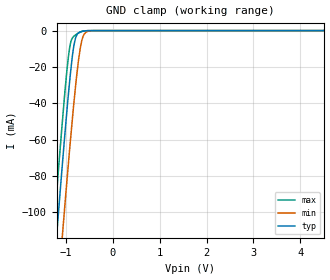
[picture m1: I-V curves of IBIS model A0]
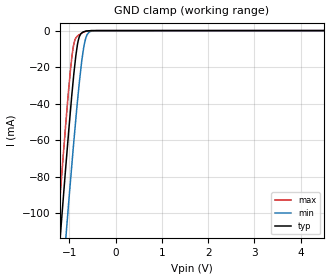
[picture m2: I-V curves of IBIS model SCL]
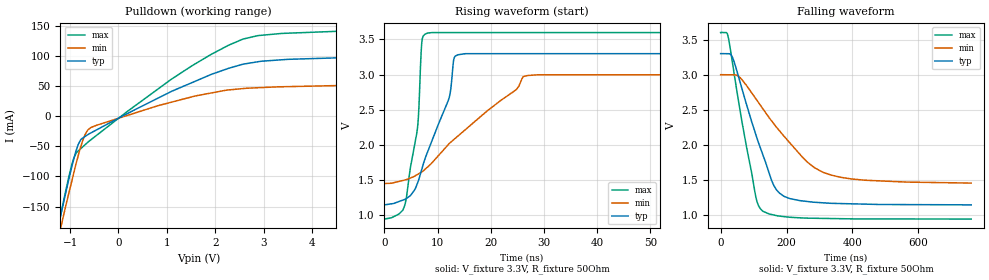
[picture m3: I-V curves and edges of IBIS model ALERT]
|Texas Instruments Incorporated
|Temperature and Supply System Monitors
|   SMBus interface
| Marketing part#   Digital Voltge  Analog Voltage   Package-type   #pins
|   Range   Range
|TMP512AIDG4   2.1V to 3.6V   3.0V to 26V   SO-14   14
|TMP512AIDRG4   2.1V to 3.6V   3.0V to 26V   SO-14   14
|TMP513AIDG4   2.1V to 3.6V   3.0V to 26V   SO-16   16
|TMP513AIDRG4   2.1V to 3.6V   3.0V to 26V   SO-16   16
|TMP513AIRSATG4   2.1V to 3.6V   3.0V to 26V   QFN-16   16
|TMP513AIRSARG4   2.1V to 3.6V   3.0V to 26V   QFN-16   16
[IBIS Ver]   4.0
[File name]   tmp512_3.ibs
[File Rev]   1.0
[Date]   04/14/2010
[Source]   Texas Instruments Incorporated.
   Analog-eLab, HPA
   12500 TI Blvd
   Dallas, TX -75243
   For Support e-mail: elab_ibis@list.ti.com
[Notes]   Revision History:
   1.0: 04/14/2010
   - Initial version of the model
   - Initial Model generated from simulations in TISPICED
   - Model not matched to measurements
   - Non-monotnic warnings - combined pulldown and pullup data
   The GPIO non-monotonic current delta is less than 1 mA in a
   full-scale range of ~95 mA. Given these conditions, these
   warnings are deemed insignificant.
   1.1: 04/18/2010 corrected spelling errors
[Disclaimer]
 This product is designed as an aid for customers of Texas Instruments.
 No warranties, either expressed or implied, with respect to this third
 party software (if any) or with respect to its fitness for any
 particular purpose is claimed by Texas Instruments or the author. The
 software (if any) is provided solely on an "as is" basis. The entire
 risk as to its quality and performance is with the customer
[Copyright] (C) Copyright 2009 Texas Instruments Incorporated.
   All rights reserved.
|   TMP512
[Component]   tmp512d   |SO-14
[Manufacturer] TI
[Package]
| variable   typ   min   max
R_pkg  0.069985   0.043420   0.089600
L_pkg  2.478174nH  1.695740nH  3.523510nH
C_pkg  0.468851pF  0.340100pF  0.678470pF
[Pin] signal_name  model_name  R_pin  L_pin C_pin
1   FILTER_C   TERM   0.04342  3.11995nH  0.67449pF
2   VP   POWER   0.08667  2.52082nH  0.46308pF
3   VINP   TERM   0.07721  2.16899nH  0.36364pF
4   VINM   TERM   0.05969  1.82032nH  0.34660pF
5   SDA   SDA   0.06085  1.85014nH  0.35048pF
6   SCL   SCL   0.08960  2.59142nH  0.46438pF
7   A0   A0   0.08471  3.52351nH  0.63150pF
8   DXP1   TERM   0.08391  3.50902nH  0.62842pF
9   DXN1   TERM   0.08732  2.54500nH  0.45919pF
10   DXP2   TERM   0.06400  1.91255nH  0.35199pF
11   DXN2   TERM   0.05307  1.69574nH  0.34010pF
12   GPIO   GPIO   0.06106  1.84901nH  0.34913pF
13   ALERT   ALERT   0.08484  2.48378nH  0.46244pF
14   GND   GND   0.04344  3.10418nH  0.6784pF
|   TMP513
[Component]   tmp513d   |SO-16
[Manufacturer] TI
[Package]
| variable   typ   min   max
R_pkg  0.065299   0.037330   0.101480
L_pkg  2.886102nH  1.773530nH  4.324090nH
C_pkg  0.858015pF  0.604310pF  1.222580pF
[Pin] signal_name  model_name  R_pin  L_pin C_pin
1   FILTER_C   TERM   0.03733  3.81993nH  1.22058pF
2   VP   POWER   0.06446  3.16263nH  0.96919pF
3   VINP   TERM   0.10148  2.80051nH  0.66655pF
4   VINM   TERM   0.07726  2.32345nH  0.63122pF
5   SDA   SDA   0.04983  1.78009nH  0.60589pF
6   SCL   SCL   0.07392  2.24087nH  0.64264pF
7   A0   A0   0.06334  3.16918nH  0.95352pF
8   DXP1   TERM   0.08068  4.32409nH  1.19594pF
9   DXN1   TERM   0.06968  4.10189nH  1.18926pF
10   DXP2   TERM   0.06456  3.19343nH  0.95660pF
11   DXN2   TERM   0.07197  2.20137nH  0.63879pF
12   DXP2   TERM   0.04946  1.77353nH  0.60431pF
13   DXN3   TERM   0.05950  1.96740nH  0.61338pF
14   GPIO   GPIO   0.08122  2.38171nH  0.64891pF
15   ALERT   ALERT   0.06271  3.12769nH  0.96888pF
16   GND   GND   0.03739  3.80986nH  1.22258pF
|   TMP513
[Component]   tmp513rsa   |QFN-16
[Manufacturer] TI
[Package]
| variable   typ   min   max
R_pkg  0.059859   0.031800   0.075880
L_pkg  1.070891nH  0.737920nH  1.352600nH
C_pkg  0.106648pF  0.097070pF  0.132860pF
[Pin] signal_name  model_name  R_pin  L_pin C_pin
1   VINP   TERM   0.07469  1.32940nH  0.11305pF
2   VINM   TERM   0.07588  1.35260nH  0.11568pF
3   SDA   SDA   0.06628  1.16760nH  0.10737pF
4   SCL   SCL   0.06192  1.08495nH  0.10230pF
5   A0   A0   0.05892  1.02585nH  0.09707pF
6   DXP1   TERM   0.06624  1.16590nH  0.10463pF
7   DXN1   TERM   0.05844  1.01645nH  0.09772pF
8   DXP2   TERM   0.06034  1.04942nH  0.09981pF
9   DXN2   TERM   0.06180  1.07436nH  0.10070pF
10   DXP3   TERM   0.06430  1.12203nH  0.10277pF
11   DXN3   TERM   0.06376  1.11165nH  0.10130pF
12   GPIO   GPIO   0.06338  1.10445nH  0.10153pF
13   ALERT   ALERT   0.05826  1.01150nH  0.09857pF
14   GND   GND   0.03196  0.73792nH  0.13286pF
15   FILTER_C   TERM   0.03180  0.73867nH  0.13120pF
16   VP   POWER   0.05978  1.04150nH  0.09980pF
|   TERM Model
[Model] TERM
Model_type Terminator
C_comp   1e-20   1e-20   1e-20
| variable   typ   min   max
[Voltage Range]   5.0V   3.3V   26V
[POWER Clamp Reference]  5.0V   3.3V   26V
[GND Clamp Reference]   0.0V   0.0V   0.0V
|Operating Temperature
[Temperature Range]   27   125   -40
| Models and submodels in the file (6): TERM (Terminator), A0 (Input), SCL (Input), ALERT (Open_drain), GPIO (I/O), SDA (I/O_open_drain)
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|   A0   3.3V digital input
[Model] A0
Model_type Input
Vinl = 0.8
Vinh = 2.1
|   typ   min   max
C_comp   1.3747800e-12   1.1549790e-12   1.6089250e-12
[Voltage Range]   3.3   3   3.6
[Temperature Range]   27   125   -40
[GND Clamp Reference]   0   0   0
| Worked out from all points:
|   GND clamp passes 1 mA (typ) near -0.72 V on its own axis
[GND Clamp]
|   Voltage   I(typ)   I(min)   I(max)
-3.3V     -841.9mA   -868mA     -829.4mA
-1.298V   -146.1mA   -184.7mA   -123.2mA
-1.247V   -129.3mA   -168mA     -106mA
-1.198V   -112.9mA   -152mA     -89.56mA
-1.089V   -77.76mA   -117mA     -54.11mA
-1.03V    -59.6mA    -98.77mA   -36.38mA
-922.3mV  -28.52mA   -65.93mA   -9.815mA
-828mV    -7.978mA   -39.34mA   -3.032mA
-706.6mV  -822.9uA   -11.99mA   -1.042mA
-612.5mV  -190.6uA   -2.027mA   -280.3uA
-420.7mV  -23.27uA   -24.62uA   -25.64uA
6.59V     0A         0A         0A
[POWER Clamp]
|   SCR cell for ESD function. Effects occurr above VDD x 2
|   Voltage   I(typ)   I(min)   I(max)
-3.3V     0A         0A         0A
0V        0A         0A         0A
6.6V      0A         0A         0A
|   SCL   3.3V digital input
[Model] SCL
Model_type Input
Vinl = 0.8
Vinh = 2.1
|   typ   min   max
C_comp   1.3747800e-12   1.1549790e-12   1.6089250e-12
[Voltage Range]   3.3   3   3.6
[Temperature Range]   27   125   -40
[GND Clamp Reference]   0   0   0
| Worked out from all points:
|   GND clamp passes 1 mA (typ) near -0.72 V on its own axis
[GND Clamp]
|   Voltage   I(typ)   I(min)   I(max)
-3.3V     -841.9mA   -868mA     -829.4mA
-1.268V   -136.1mA   -174.8mA   -113mA
-1.213V   -118mA     -156.9mA   -94.64mA
-1.172V   -104.6mA   -143.8mA   -81.14mA
-1.081V   -75.19mA   -114.5mA   -51.62mA
-1.028V   -58.9mA    -98.01mA   -35.65mA
-939.6mV  -33.06mA   -71.14mA   -12.97mA
-821.2mV  -7.015mA   -37.56mA   -2.864mA
-706.5mV  -822uA     -11.97mA   -986.9uA
-614.8mV  -199.1uA   -2.129mA   -274.3uA
-414.7mV  -19.06uA   -20.97uA   -26.82uA
6.59V     0A         0A         0A
[POWER Clamp]
|   SCR cell for ESD function. Effects occurr above VDD x 2
|   Voltage   I(typ)   I(min)   I(max)
-3.3V     0A         0A         0A
0V        0A         0A         0A
6.6V      0A         0A         0A
|   ALERT  3.3V digital open_drain_output
[Model] ALERT
Model_type Open_drain
Polarity   Non-Inverting
Enable   Active-Low
Vmeas = 1.55
Vref = 1.55
Cref = 15pF
Rref = 50
|   typ   min   max
|   average of high and low
C_comp   3.14511E-11   2.22383E-11   4.79695E-11
|   output high
|C_comp   6.0547790e-11   4.1719200e-11   9.3964360e-11
|   output low
|C_comp   2.3544370e-12   1.9745760e-12   2.7573970e-12
[Voltage Range]   3.3   3   3.6
[Temperature Range]   27   125   -40
[GND Clamp Reference]   0   0   0
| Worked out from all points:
|   slope of the pulldown table from 0 to 0.495 V, typ, clamps not added: 24.5 ohm
|   falling waveform, V_fixture 3.3V, R_fixture 50Ohm: 20-80 % time 88.2ns typ, 159ns min, 59.5ns max; typ from 3.3 V to 1.15 V
|   rising waveform, V_fixture 3.3V, R_fixture 50Ohm: 20-80 % time 5.85ns typ, 13.8ns min, 2.23ns max; typ from 1.15 V to 3.3 V
[Pulldown]
|   Voltage   I(typ)   I(min)   I(max)
-3.3V     -1.009A    -981.4mA   -1.084A
-1.26V    -188.9mA   -208.4mA   -188.9mA
-1.158V   -151.1mA   -172.4mA   -149.4mA
-923.4mV  -70.83mA   -93.78mA   -69.44mA
-833.4mV  -47.04mA   -65.7mA    -57.65mA
-742mV    -36.33mA   -40.97mA   -51.04mA
-642.6mV  -31.1mA    -23.79mA   -43.85mA
-568.7mV  -27.64mA   -18.81mA   -39mA
1.104V    41.42mA    23.4mA     61.79mA
2.563V    85.92mA    45.68mA    127.5mA
3.371V    93.46mA    48.74mA    137.2mA
6.59V     101.8mA    54.33mA    147.1mA
[Ramp]
R_load = 50
|   typ   min   max
dV/dt_r   1.29119/5.84006e-009   0.929/1.37888e-008   1.59202/2.23001e-009
dV/dt_f   1.29085/8.79694e-008  0.925043/1.59373e-007   1.592/5.96441e-008
[Falling Waveform]
V_fixture = 3.3V
V_fixture_min = 3V
V_fixture_max = 3.6V
R_fixture = 50Ohm
C_fixture = 0F
|   Time   V(typ)   V(min)   V(max)
0s        3.3V       3V         3.6V
22.44ns   3.298V     2.999V     3.549V
40.54ns   3.189V     2.998V     3.03V
105.9ns   2.162V     2.664V     1.283V
127.5ns   1.869V     2.52V      1.06V
154.9ns   1.494V     2.341V     1.011V
178.6ns   1.316V     2.202V     988.6mV
262.4ns   1.197V     1.76V      959.6mV
313.4ns   1.177V     1.607V     955.7mV
760.2ns   1.149V     1.458V     946.7mV
[Rising Waveform]
V_fixture = 3.3V
V_fixture_min = 3V
V_fixture_max = 3.6V
R_fixture = 50Ohm
C_fixture = 0F
|   Time   V(typ)   V(min)   V(max)
0s        1.148V     1.452V     946.6mV
3.922ns   1.228V     1.503V     1.162V
6.296ns   1.468V     1.583V     2.284V
7.116ns   1.672V     1.62V      3.503V
8.925ns   2.054V     1.743V     3.598V
12.2ns    2.675V     2.02V      3.598V
13.14ns   3.242V     2.082V     3.598V
15.23ns   3.298V     2.218V     3.598V
28.85ns   3.298V     2.998V     3.598V
760.2ns   3.3V       3V         3.6V
